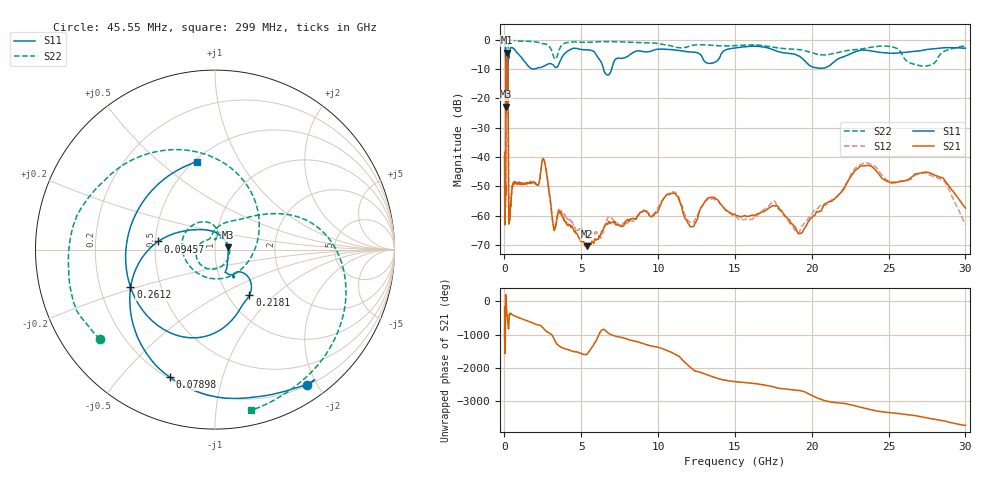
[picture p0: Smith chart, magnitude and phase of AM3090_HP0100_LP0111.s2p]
! Date/Time: Thu, Feb 28, 2019 1:57 PM
! Network Analyzer: Agilent Technologies E8364B Rev: A.07.50.67
! Sweep from 0.010 to 30.000 GHz, 1601 Points, Sweep Type: LOG
! Power Supply: 5.023 V, 0.002 A
# Hz S DB R 50
!freq MagS11 AngS11 MagS21 AngS21 MagS12 AngS12 MagS22 AngS22
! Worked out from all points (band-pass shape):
!   1601 points, 10 MHz to 30 GHz, reference 50 ohm
!   highest |S21| = -4.31 dB at 153.7 MHz (marker M1); lowest = -70.4 dB at 5.365 GHz (marker M2)
!   |S21| within 3 dB of the highest: 105.9 MHz to 217.2 MHz (111.3 MHz wide, 68.9 % of centre)
!   lowest |S11| = -22.8 dB at 103.5 MHz (marker M3), VSWR 1.16, Z = 57.7 + j1.45 ohm
!   |S11| at or under -10 dB: 94.64 MHz to 217.7 MHz (123.1 MHz wide, 78.8 % of centre); 6.455 GHz to 6.978 GHz (522.7 MHz wide, 7.78 % of centre)
!   |S22| runs from -25.2 to -0.2 dB; largest |S21 - S12| = 0.011
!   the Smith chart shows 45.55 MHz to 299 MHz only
!   S11 on the Smith chart (normalised r, x): 45.55 MHz: 0.21, -1.87; 78.98 MHz: 0.21, -0.69; 94.57 MHz: 0.52, +0.05; 218.1 MHz: 1.25, -0.71; 261.2 MHz: 0.33, -0.19; 299 MHz: 0.52, +0.68
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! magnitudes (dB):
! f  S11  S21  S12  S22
! 10 MHz  -0.2  -38.3  -39.5  -0.6
! 38.04 MHz  -0.5  -60.3  -59.5  -1.4
! 45.55 MHz  -0.8  -56.6  -55.0  -1.8
! 78.98 MHz  -2.5  -48.3  -48.8  -4.7
! 94.57 MHz  -9.9  -16.8  -16.9  -15.6
! 103.5 MHz  -22.8  -8.2  -8.2  -14.4
! 144.7 MHz  -15.7  -4.4  -4.3  -22.4
! 153.7 MHz  -15.4  -4.3  -4.3  -21.4
! 218.1 MHz  -9.9  -7.5  -7.5  -15.9
! 236.3 MHz  -7.6  -16.3  -16.3  -8.4
! 261.2 MHz  -5.8  -48.4  -47.8  -1.8
! 299 MHz  -6.0  -60.7  -60.4  -0.7
! 550.5 MHz  -2.8  -49.4  -49.0  -0.3
! 2.084 GHz  -9.8  -49.4  -49.2  -0.7
! 2.558 GHz  -9.0  -40.8  -40.6  -1.3
! 3.236 GHz  -8.9  -65.1  -64.4  -6.2
! 5.365 GHz  -3.4  -70.4  -66.7  -0.8
! 7.926 GHz  -5.9  -61.8  -62.7  -0.7
! 10.86 GHz  -3.3  -52.4  -51.9  -2.0
! 19.22 GHz  -5.6  -66.1  -65.3  -3.3
! 23.48 GHz  -3.5  -43.0  -42.0  -2.9
! 30 GHz  -2.8  -57.4  -63.0  -2.2
